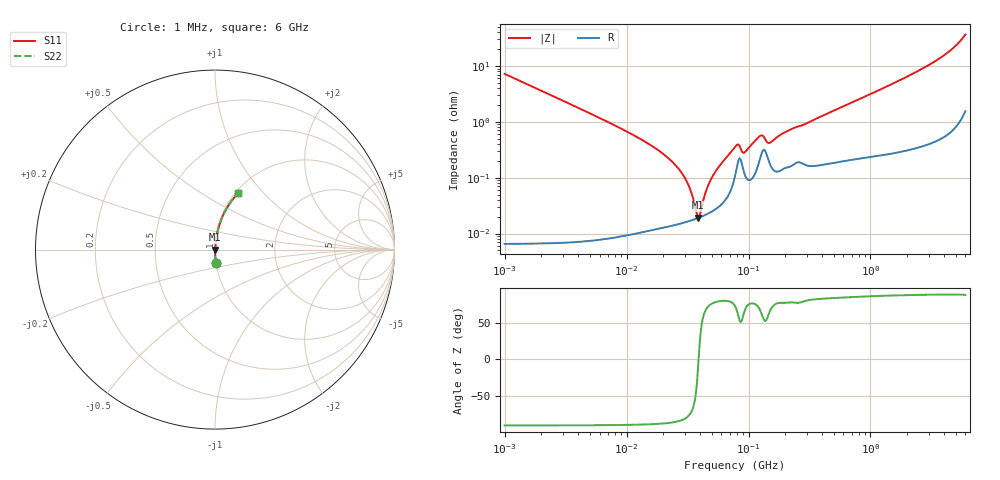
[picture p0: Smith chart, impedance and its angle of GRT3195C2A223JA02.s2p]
!Murata Part Number: GRT3195C2A223JA02
!These Parameters are Measured in Series Mode Connection
!Data Generated on Jun 19, 2026
!  o--ll--o
!Port1  Port2
!  o------o
!Operation Temp=25[degC], DC Bias Voltage=0[V]
!Freq. Start=1000[kHz] Stop=6[GHz] 401[Steps]
# Hz S RI R 50
!Freq.(Hz) S11(Real) S11(Imag) S21(Real) S21(Imag) S12(Real) S12(Imag) S22(Real) S22(Imag)
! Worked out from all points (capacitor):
!   401 points, 1 MHz to 6 GHz, reference 50 ohm
!   read as one part in series: C = 22 nF near 1.044 MHz
!   lowest |Z| = 19.3 mohm at 38.62 MHz (marker M1)
!   series resonance near 38.97 MHz, so ESL is about 760 pH
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1000000  0.00526 -0.0719  0.9947 0.0719  0.9947 0.0719  0.00526 -0.0719
4293785  0.000348 -0.0166  0.9997 0.0166  0.9997 0.0166  0.000348 -0.0166
1.0704e7  0.000134 -0.00623  0.9999 0.00623  0.9999 0.00623  0.000134 -0.00623
1.843659e7  0.000131 -0.00304  0.9999 0.00304  0.9999 0.00304  0.000131 -0.00304
2.393455e7  0.000143 -0.00188  0.9999 0.00188  0.9999 0.00188  0.000143 -0.00188
2.910942e7  0.000157 -0.0011  0.9998 0.0011  0.9998 0.0011  0.000157 -0.0011
3.316698e7  0.00017 -0.000605  0.9998 0.000605  0.9998 0.000605  0.00017 -0.000605
3.697709e7  0.000184 -0.000197  0.9998 0.000197  0.9998 0.000197  0.000184 -0.000197
3.8621e7  0.00019 -3.34e-05  0.9998 3.34e-05  0.9998 3.34e-05  0.00019 -3.34e-05
4.033799e7  0.000198 0.000131  0.9998 -0.000131  0.9998 -0.000131  0.000198 0.000131
4.497189e7  0.00022 0.000547  0.9998 -0.000547  0.9998 -0.000547  0.00022 0.000547
5.013812e7  0.00025 0.000981  0.9998 -0.000981  0.9998 -0.000981  0.00025 0.000981
7.745967e7  0.00108 0.00338  0.9989 -0.00338  0.9989 -0.00338  0.00108 0.00338
8.268215e7  0.00206 0.00333  0.9979 -0.00333  0.9979 -0.00333  0.00206 0.00333
9.218041e7  0.00123 0.00252  0.9988 -0.00252  0.9988 -0.00252  0.00123 0.00252
1.249896e8  0.00231 0.00513  0.9977 -0.00513  0.9977 -0.00513  0.00231 0.00513
1.487431e8  0.00184 0.00377  0.9982 -0.00377  0.9982 -0.00377  0.00184 0.00377
1.973453e8  0.00151 0.00627  0.9985 -0.00627  0.9985 -0.00627  0.00151 0.00627
3.325952e8  0.00172 0.0103  0.9983 -0.0103  0.9983 -0.0103  0.00172 0.0103
1.428092e9  0.00465 0.0447  0.9953 -0.0447  0.9953 -0.0447  0.00465 0.0447
3.5601e9  0.0211 0.1269  0.9789 -0.1269  0.9789 -0.1269  0.0211 0.1269
6e9  0.1284 0.3139  0.8716 -0.3139  0.8716 -0.3139  0.1284 0.3139
